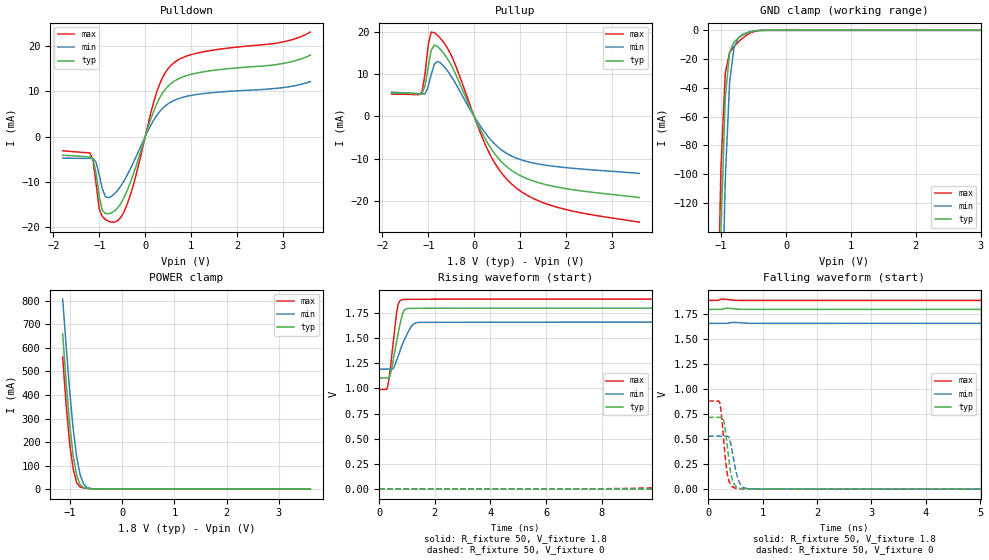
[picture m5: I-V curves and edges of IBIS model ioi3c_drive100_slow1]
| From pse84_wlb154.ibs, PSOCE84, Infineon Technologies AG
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[Model] ioi3c_drive100_slow1
Model_type I/O
Enable   Active-High
Vinl  =  0.54
Vinh  =  1.26
Vmeas =  0.9
Cref  =  15e-12
| Capacitance   typ   min   max
C_comp   9.12545e-13 8.87504e-13 9.42456e-13
| Variables   typ   min   max
[GND Clamp Reference]   0   0   0
[POWER Clamp Reference]   1.8   1.66   1.89
[Pulldown Reference]   0   0   0
[Pullup Reference]   1.8   1.66   1.89
[Temperature Range]   25   125   -40
[Voltage Range]   1.8   1.66   1.89
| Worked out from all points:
|   slope of the pulldown table from 0 to 0.27 V, typ, clamps not added: 35.5 ohm
|   slope of the pullup table from 0 to 0.27 V, typ, clamps not added: 46.2 ohm
|   GND clamp passes 1 mA (typ) near -0.55 V on its own axis
|   POWER clamp passes 1 mA (typ) near -0.54 V on its own axis
|   falling waveform, R_fixture 50, V_fixture 1.8: 20-80 % time 82.7ns typ, 123ns min, 48.8ns max; typ from 1.8 V to 1.1 V
|   falling waveform, R_fixture 50, V_fixture 0: 20-80 % time 103ps typ, 120ps min, 94.3ps max; typ from 0.72 V to 0 V
|   rising waveform, R_fixture 50, V_fixture 1.8: 20-80 % time 285ps typ, 412ps min, 221ps max; typ from 1.1 V to 1.8 V
|   rising waveform, R_fixture 50, V_fixture 0: 20-80 % time 90.2ns typ, 134ns min, 54.8ns max; typ from 0 V to 0.72 V
[GND Clamp]
| Voltage   I(typ)   I(min)   I(max)
-1.204V   -737.9mA   -831.5mA   -678.7mA
-1.07V    -303.2mA   -410.8mA   -239.8mA
-1.003V   -139.9mA   -232.2mA   -95.74mA
-936.6mV  -46.51mA   -103.5mA   -29.5mA
-869.7mV  -15.31mA   -35.88mA   -15.36mA
-802.8mV  -8.166mA   -12.13mA   -11.29mA
-735.9mV  -5.335mA   -5.292mA   -8.195mA
-669mV    -3.356mA   -2.85mA    -5.457mA
-535.2mV  -837.9uA   -772uA     -1.483mA
-401.4mV  -47.36uA   -84.85uA   -76.77uA
3.6V      0A         0A         0A
[POWER Clamp]
| Voltage   I(typ)   I(min)   I(max)
-1.137V   660mA      807.5mA    561.8mA
-1.07V    454.5mA    608.2mA    356.2mA
-1.003V   275.7mA    418.4mA    193.6mA
-936.6mV  143.5mA    257.2mA    86.91mA
-869.7mV  59.43mA    137.9mA    27.31mA
-802.8mV  18.8mA     60.93mA    8.704mA
-735.9mV  6.231mA    21.35mA    5.155mA
-669mV    3.127mA    6.887mA    3.44mA
-535.2mV  940.9uA    1.232mA    1.058mA
-334.5mV  16.1uA     59.03uA    7.686uA
3.6V      0A         0A         0A
[Pulldown]
| Voltage   I(typ)   I(min)   I(max)
-1.8V     -4.088mA   -4.719mA   -3.118mA
-1.204V   -4.463mA   -4.803mA   -3.601mA
-1.137V   -4.911mA   -4.804mA   -5.306mA
-1.003V   -13.12mA   -8.336mA   -15.89mA
-936.6mV  -16.2mA    -11.45mA   -17.55mA
-802.8mV  -16.98mA   -13.46mA   -18.62mA
-602.1mV  -15.71mA   -11.83mA   -18.51mA
-267.6mV  -8.526mA   -5.918mA   -10.98mA
248.3mV   7.148mA    4.62mA     9.711mA
558.6mV   11.66mA    7.598mA    15.64mA
1.117V    13.97mA    9.25mA     18.34mA
3.6V      17.92mA    12.1mA     23mA
[Pullup]
| Voltage   I(typ)   I(min)   I(max)
-1.8V     5.566mA    5.757mA    5.298mA
-1.137V   5.423mA    5.336mA    5.817mA
-1.07V    7.237mA    5.348mA    10.12mA
-1.003V   11.65mA    7.007mA    16.92mA
-936.6mV  15.64mA    9.959mA    19.98mA
-869.7mV  16.91mA    12.35mA    19.85mA
-735.9mV  15.89mA    12.69mA    18.5mA
-468.3mV  11.47mA    8.972mA    13.74mA
310.3mV   -6.605mA   -4.872mA   -8.255mA
806.9mV   -12.71mA   -9.338mA   -15.91mA
1.738V    -16.58mA   -11.8mA    -21.28mA
3.6V      -19.2mA    -13.5mA    -25.05mA
[Ramp]
dV/dt_r   0.431994/90.1718n  0.318355/0.13411u  0.529893/54.7532n
dV/dt_f   0.41826/82.7113n  0.280676/0.123121u  0.54002/48.8334n
R_load = 50
[Falling Waveform]
R_fixture = 50
V_fixture = 1.8
V_fixture_min = 1.66
V_fixture_max = 1.89
| Time   V(typ)   V(min)   V(max)
0s        1.8V       1.66V      1.89V
8.73ns    1.8V       1.66V      1.873V
17.67ns   1.777V     1.659V     1.719V
31.97ns   1.667V     1.635V     1.486V
56.52ns   1.485V     1.552V     1.234V
81.59ns   1.352V     1.468V     1.107V
123.4ns   1.224V     1.363V     1.025V
189.4ns   1.142V     1.272V     995.5mV
303.2ns   1.109V     1.213V     990.2mV
800ns     1.103V     1.192V     990mV
[Falling Waveform]
R_fixture = 50
V_fixture = 0
V_fixture_min = 0
V_fixture_max = 0
| Time   V(typ)   V(min)   V(max)
0s        720mV      530.8mV    883.2mV
212.1ps   719.8mV    530.8mV    864.3mV
240.2ps   720.1mV    530.8mV    763.2mV
282.3ps   694.8mV    530.7mV    508.9mV
342.5ps   460.5mV    531mV      184.5mV
428.7ps   124.6mV    415.1mV    33.87mV
538.6ps   16.63mV    119.2mV    6.466mV
638.8ps   4.684mV    20.99mV    2.996mV
1.499ns   1.137mV    1.006mV    1.325mV
800ns     11.39nV    753.4nV    4.342nV
[Rising Waveform]
R_fixture = 50
V_fixture = 1.8
V_fixture_min = 1.66
V_fixture_max = 1.89
| Time   V(typ)   V(min)   V(max)
0s        1.103V     1.192V     990mV
302ps     1.103V     1.192V     1.02V
415.4ps   1.157V     1.192V     1.24V
613.8ps   1.452V     1.269V     1.728V
718.1ps   1.602V     1.353V     1.862V
856.1ps   1.755V     1.453V     1.885V
954ps     1.79V      1.514V     1.887V
1.297ns   1.798V     1.651V     1.888V
1.799ns   1.799V     1.659V     1.889V
800ns     1.8V       1.66V      1.89V
[Rising Waveform]
R_fixture = 50
V_fixture = 0
V_fixture_min = 0
V_fixture_max = 0
| Time   V(typ)   V(min)   V(max)
0s        11.38nV    752.4nV    4.339nV
11.02ns   214.7uV    -179.3uV   20.71mV
20.37ns   29.28mV    3.362mV    158mV
37.24ns   153.9mV    42.7mV     399.2mV
65.3ns    344.7mV    146.5mV    649.3mV
90.38ns   466.4mV    230.9mV    760.7mV
132.2ns   588.8mV    337mV      839.9mV
201.1ns   674.9mV    437.7mV    874.8mV
312.4ns   711.6mV    502.1mV    882.5mV
800ns     720mV      530.6mV    883.2mV
